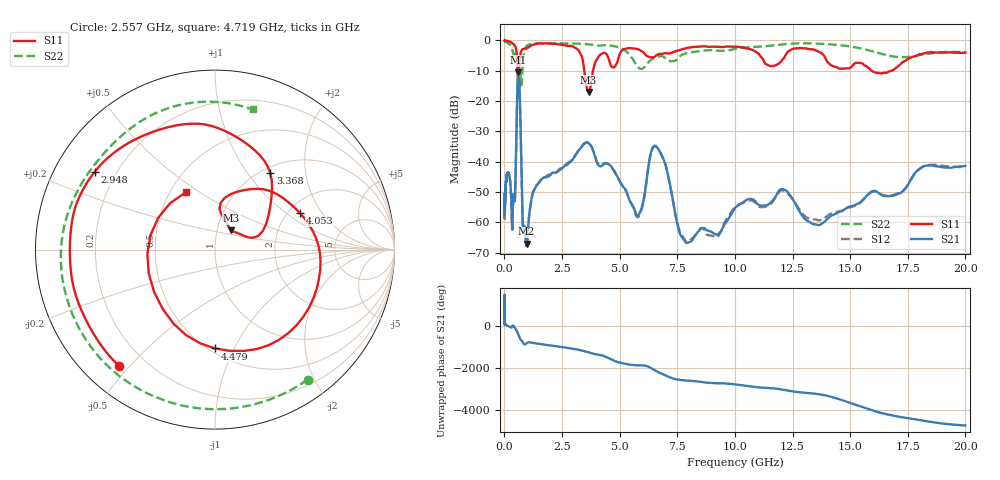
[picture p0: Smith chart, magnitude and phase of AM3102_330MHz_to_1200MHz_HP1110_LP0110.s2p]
! Date/Time: Tue, Sep 11, 2018 5:23 PM
! Network Analyzer: Agilent Technologies E8362B Rev: A.07.50.63
! Sweep from 0.010 to 20.000 GHz, 1601 Points, Sweep Type: LOG
! Power Supply: 4.949 V, 0.001 A
# Hz S DB R 50
!freq MagS11 AngS11 MagS21 AngS21 MagS12 AngS12 MagS22 AngS22
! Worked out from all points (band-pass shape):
!   1601 points, 10 MHz to 20 GHz, reference 50 ohm
!   highest |S21| = -10.52 dB at 609 MHz (marker M1); lowest = -67.1 dB at 965.5 MHz (marker M2)
!   |S21| within 3 dB of the highest: 575.8 MHz to 644.5 MHz (68.67 MHz wide, 11.3 % of centre)
!   lowest |S11| = -17.1 dB at 3.651 GHz (marker M3), VSWR 1.33, Z = 58.4 + j12.8 ohm
!   |S11| at or under -10 dB: 570.3 MHz to 635.4 MHz (65.06 MHz wide, 10.8 % of centre); 3.467 GHz to 3.846 GHz (378.5 MHz wide, 10.4 % of centre); 15.92 GHz to 16.8 GHz (885.6 MHz wide, 5.41 % of centre)
!   |S22| runs from -15.8 to -0.2 dB; largest |S21 - S12| = 0.0055
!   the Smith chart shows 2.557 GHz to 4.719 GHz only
!   S11 on the Smith chart (normalised r, x): 2.557 GHz: 0.11, -0.47; 2.948 GHz: 0.12, +0.29; 3.368 GHz: 1.09, +1.29; 4.053 GHz: 2.30, +1.28; 4.479 GHz: 0.53, -0.84; 4.719 GHz: 0.60, +0.44
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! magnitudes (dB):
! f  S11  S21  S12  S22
! 10 MHz  0.0  -50.7  -59.0  -0.2
! 35.55 MHz  -0.1  -51.6  -50.6  -0.4
! 126.4 MHz  -0.2  -44.1  -44.0  -0.8
! 254.1 MHz  -0.5  -46.4  -46.8  -1.5
! 337.9 MHz  -1.0  -62.4  -62.0  -3.0
! 447.2 MHz  -1.8  -53.1  -52.3  -4.2
! 609 MHz  -13.7  -10.5  -10.6  -15.4
! 676.1 MHz  -5.6  -20.3  -20.3  -10.7
! 798.4 MHz  -2.9  -60.4  -61.6  -7.8
! 965.5 MHz  -2.7  -67.1  -67.6  -1.9
! 1.59 GHz  -1.1  -45.9  -46.0  -1.0
! 2.557 GHz  -1.5  -41.9  -41.9  -1.0
! 2.948 GHz  -2.0  -39.5  -39.2  -1.0
! 3.368 GHz  -5.6  -34.9  -35.0  -1.2
! 3.651 GHz  -17.1  -33.9  -33.7  -1.3
! 4.053 GHz  -5.8  -40.9  -40.6  -1.7
! 4.479 GHz  -5.2  -40.7  -40.6  -1.6
! 4.719 GHz  -8.9  -42.5  -42.6  -1.9
! 5.652 GHz  -2.7  -56.0  -56.4  -7.2
! 6.58 GHz  -5.0  -34.9  -35.1  -5.5
! 7.958 GHz  -2.5  -66.8  -66.4  -4.2
! 20 GHz  -4.0  -41.4  -41.9  -3.9
